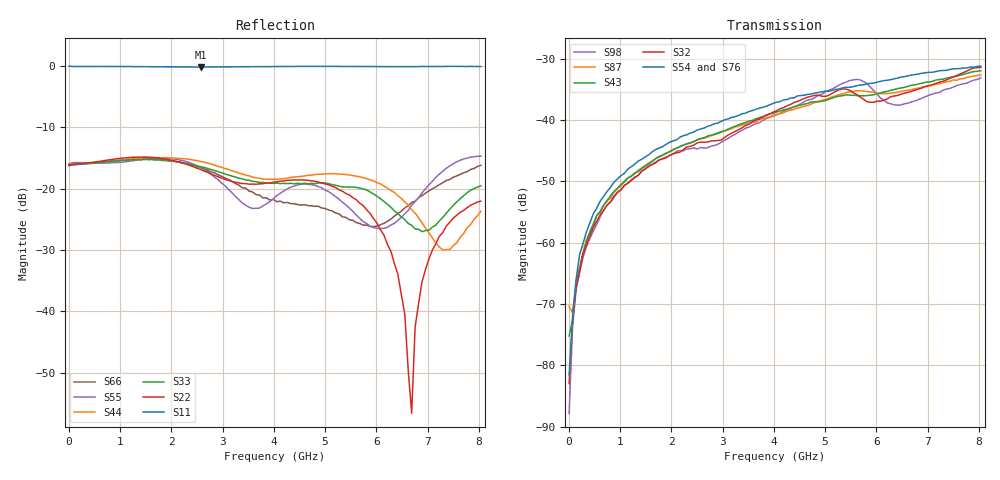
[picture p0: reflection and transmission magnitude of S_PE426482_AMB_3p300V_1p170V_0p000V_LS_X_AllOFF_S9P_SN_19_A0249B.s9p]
! Device ID: PE426482
! File Path: z:\PE426482\All_Of_State_PE426482\Re-Measure\AMB\3p300\LS_X\PE426482_AMB_3p300V_1p170V_0p000V_LS_X_AllOFF_S9P_SN_19_A0249B.s9p
! Serial: 19
! Lot: A0249B
! Temp: AMB
! VDD: 3.300
! VSS: 0.000
! Control_Hi: 1.170
! Control_Lo: 0.000
! Logic State: LS_X_AllOFF
! Port 1:
! Port 2:
! Port 3:
! Port 4:
! Port 5:
! Port 6:
! Port 7:
! Port 8:
! Port 9:
! ThroughPath:1-2
! IDD: 0.000106564
! ISS/IDD2: 0
! IDMM3/IDD3: -1.572e-007
! Comment:
#  Hz  S  RI  R  50
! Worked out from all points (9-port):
!   120 points, 10 MHz to 8.037 GHz, reference 50 ohm
!   strongest paths, dB at 10 MHz, 2.034 GHz, 4.057 GHz, 6.08 GHz, 8.037 GHz:
!     S54: -81.5, -43.4, -37.1, -33.7, -31.2
!     S76: -80.8, -43.2, -37.5, -33.6, -31.1
!     S32: -82.9, -45.5, -38.5, -36.9, -31.4
!     S43: -75.2, -44.9, -38.7, -35.6, -32.0
!     S87: -70.3, -44.7, -39.0, -35.7, -32.6
!     S98: -87.8, -45.5, -39.2, -36.4, -33.1
!   lowest |S11| = -0.2 dB at 2.573 GHz (marker M1), VSWR 115.29, Z = 0.435 - j2.38 ohm
!   |S11| at or under -10 dB: nowhere
